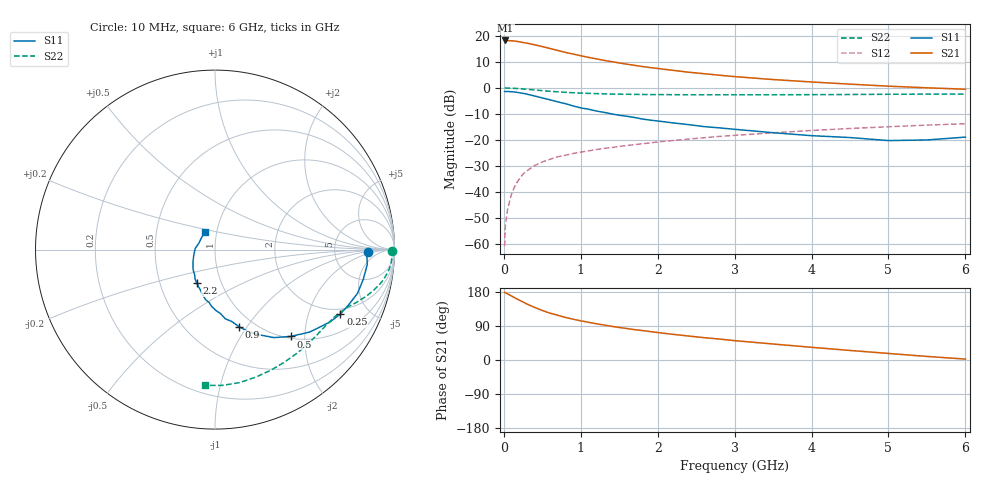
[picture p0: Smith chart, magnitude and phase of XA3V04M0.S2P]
! SIEMENS Discrete & RF Semiconductors
! BFY180
! Si NPN RF Bipolar Junction Transistor in MICRO-X
! VCE = 3 V  IC = 4 mA
! Common Emitter S-Parameters:  May  1997
# GHz  S  MA  R  50
!  f  S11  S21  S12  S22
! GHz  MAG  ANG  MAG  ANG  MAG  ANG  MAG  ANG
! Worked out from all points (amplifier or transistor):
!   36 points, 10 MHz to 6 GHz, reference 50 ohm
!   highest |S21| = 18.2 dB at 20 MHz (marker M1)
!   |S21| within 3 dB of that: start of sweep to 588.1 MHz
!   unconditionally stable (mu >= 1): 1.547 GHz to end of sweep
!   at 250 MHz: K = 0.24, MSG = 25.3 dB, |S12| = -33.2 dB
!   at 1.4 GHz: K = 0.97, MSG = 16.5 dB, |S12| = -23.0 dB
!   at 6 GHz: K = 1.10, MAG = 4.7 dB, |S12| = -13.8 dB
!   S11 on the Smith chart (normalised r, x): 10 MHz: 13, -1; 250 MHz: 1.74, -3.27; 500 MHz: 1.03, -1.70; 900 MHz: 0.85, -0.92; 2.2 GHz: 0.76, -0.30; 6 GHz: 0.88, +0.17
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0.01  0.8542 -1.0  8.099 178.6  0.0009 83.3  0.9888 -0.3
0.02  0.847 -2.0  8.173 177.4  0.0023 94.0  0.9941 -0.7
0.05  0.8522 -5.6  8.079 174.4  0.0047 87.9  0.988 -2.1
0.1  0.8428 -11.3  8.055 168.9  0.0091 84.4  0.984 -4.3
0.15  0.8303 -17.1  7.91 163.3  0.0136 80.4  0.9773 -6.3
0.25  0.7852 -27.2  7.457 153.0  0.022 75.4  0.9538 -10.1
0.3  0.757 -32.2  7.267 147.8  0.0253 72.6  0.9396 -11.7
0.4  0.6993 -41.1  6.741 138.8  0.0321 68.3  0.9111 -14.5
0.5  0.6412 -49.0  6.233 130.7  0.0375 64.3  0.8845 -16.9
0.6  0.59 -56.2  5.728 123.6  0.0423 61.9  0.8595 -18.9
0.7  0.5384 -62.1  5.254 118.2  0.0472 59.3  0.8398 -20.6
0.8  0.4966 -67.5  4.817 112.3  0.0506 57.9  0.8204 -22.1
0.9  0.45 -72.7  4.474 107.7  0.0546 56.6  0.8058 -23.4
1.1  0.3898 -81.5  3.864 99.6  0.0613 55.0  0.7834 -26.1
1.5  0.2971 -96.2  3.02 85.8  0.0746 52.4  0.7571 -31.4
1.7  0.2692 -103.5  2.713 80.1  0.0807 51.6  0.7484 -34.0
2.2  0.2118 -119.0  2.174 67.7  0.0972 49.0  0.7405 -40.9
2.8  0.1701 -134.8  1.753 55.3  0.1162 45.3  0.7359 -49.0
3.5  0.1372 -153.0  1.446 42.2  0.1366 40.6  0.7368 -58.5
4.5  0.1107 176.9  1.18 25.2  0.1653 33.1  0.7459 -72.2
5.5  0.0995 140.0  1.003 9.4  0.1921 25.4  0.7576 -86.8
6  0.1129 120.1  0.942 2.4  0.2044 21.0  0.7586 -94.1
